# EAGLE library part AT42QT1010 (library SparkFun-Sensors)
Atmel AT42QT1010 The AT42QT1010 (QT1010) is a digital burst mode charge-transfer (QT™) sensor that is capable of detecting nearproximityor touch, making it ideal for implementing touch controls.The QT1010 is designed specifically for human interfaces, like control panels, appliances, toys, lighting controls, or anywhere a mechanical switch or button may be found. It includes all hardware and signal processing functions necessary to provide stable sensing under a wide variety of changing conditions. Only a single low-cost capacitor is required for operation. Datasheet Sparkfun Products Sparkfun Capacitive Touch Breakout (SEN-12041)
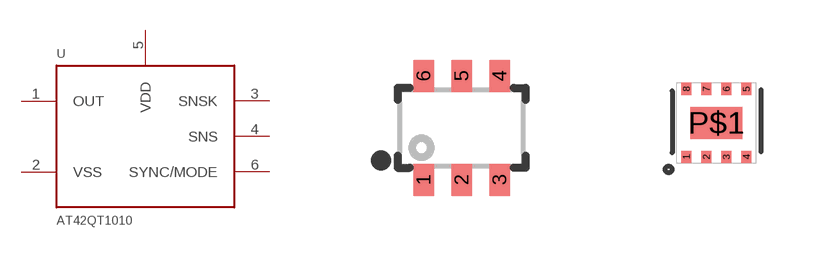
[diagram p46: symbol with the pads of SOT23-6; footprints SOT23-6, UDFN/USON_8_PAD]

Designator prefix -

## AT42QT1010SOT23  [SOT23-6]
1  OUT
2  VSS
3  SNSK
4  SNS
5  VDD
6  SYNC/MODE

## AT42QT1010UDFN (PROD_ID: IC-13773; VALUE: AT42QT1010 - UDFN)  [UDFN/USON_8_PAD]
1  SNSK
4  VSS
5  OUT
6  SYNC/MODE
7  VDD
8  SNS

## Footprint SOT23-6 (pad centres in mm)
6-Pin SOT23-6 Datasheet Specifications: Pin Count: 6 Area: 2.6 x 2.9 x 1.45 mm Pitch: 0.95 mm Devices Using: AT42QT1012
smd 0.51 x 0.8: 1 -0.95,-1.3; 2 0,-1.3; 3 0.95,-1.3; 4 0.95,1.3; 5 0,1.3; 6 -0.95,1.3

## Footprint UDFN/USON_8_PAD (pad centres in mm)
smd 0.25 x 0.3: 1 -0.75,-0.852; 2 -0.25,-0.852; 3 0.25,-0.852; 4 0.75,-0.852; 5 0.75,0.852; 6 0.25,0.852; 7 -0.25,0.852; 8 -0.75,0.852
smd 1.3 x 0.8: P$1 0,0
